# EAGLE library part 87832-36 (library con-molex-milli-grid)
HEADER
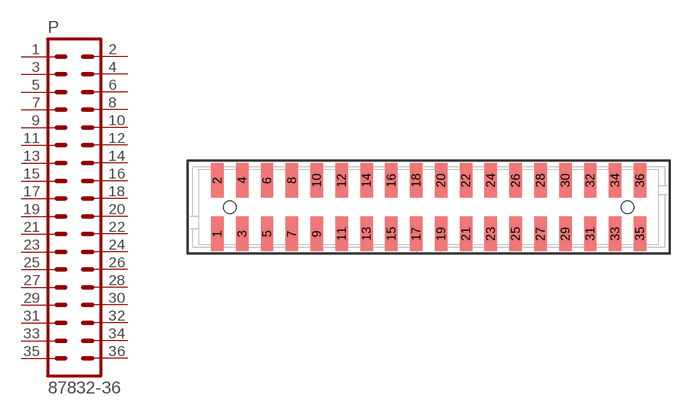
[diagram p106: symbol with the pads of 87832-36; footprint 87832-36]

Designator prefix P

## 87832-36  [87832-36]
1  1  pas
2  2  pas
3  3  pas
4  4  pas
5  5  pas
6  6  pas
7  7  pas
8  8  pas
9  9  pas
10  10  pas
11  11  pas
12  12  pas
13  13  pas
14  14  pas
15  15  pas
16  16  pas
17  17  pas
18  18  pas
19  19  pas
20  20  pas
21  21  pas
22  22  pas
23  23  pas
24  24  pas
25  25  pas
26  26  pas
27  27  pas
28  28  pas
29  29  pas
30  30  pas
31  31  pas
32  32  pas
33  33  pas
34  34  pas
35  35  pas
36  36  pas

## Footprint 87832-36 (pad centres in mm)
HEADER SMD Dual Row, Shrouded, Vertical
smd 1 x 2.75: 1 -17,-2.15; 2 -17,2.15; 3 -15,-2.15; 4 -15,2.15; 5 -13,-2.15; 6 -13,2.15; 7 -11,-2.15; 8 -11,2.15; 9 -9,-2.15; 10 -9,2.15; 11 -7,-2.15; 12 -7,2.15; 13 -5,-2.15; 14 -5,2.15; 15 -3,-2.15; 16 -3,2.15; 17 -1,-2.15; 18 -1,2.15; 19 1,-2.15; 20 1,2.15; 21 3,-2.15; 22 3,2.15; 23 5,-2.15; 24 5,2.15; 25 7,-2.15; 26 7,2.15; 27 9,-2.15; 28 9,2.15; 29 11,-2.15; 30 11,2.15; 31 13,-2.15; 32 13,2.15; 33 15,-2.15; 34 15,2.15; 35 17,-2.15; 36 17,2.15
hole 1 at -16,0
hole 1 at 16,0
